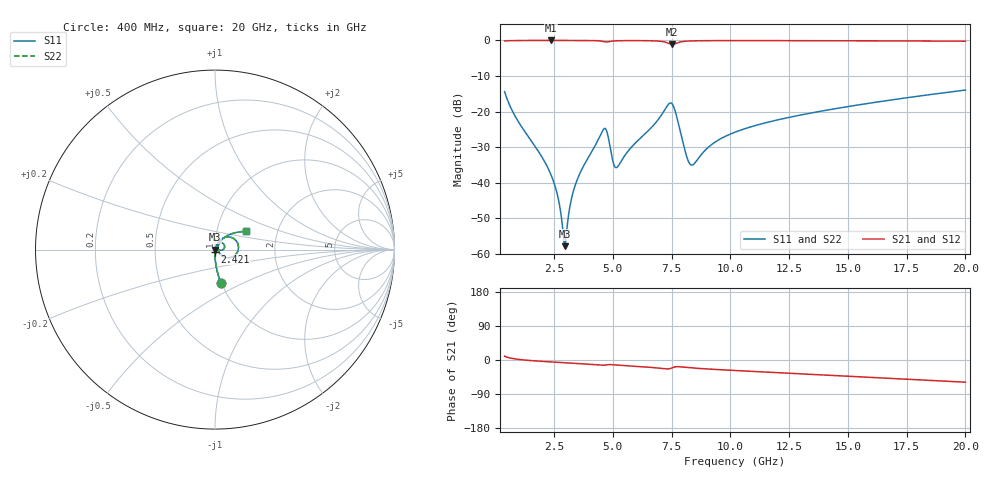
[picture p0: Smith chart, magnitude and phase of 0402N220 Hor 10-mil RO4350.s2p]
# GHz S MA R 50
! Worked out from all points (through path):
!   1960 points, 400 MHz to 20 GHz, reference 50 ohm
!   highest |S21| = -0.01 dB at 2.371 GHz (marker M1); lowest = -1.1 dB at 7.534 GHz (marker M2)
!   group delay of S21, straight-line fit = 8.43 ps
!   lowest |S11| = -57.9 dB at 2.961 GHz (marker M3), VSWR 1.00, Z = 50.1 - j0.0167 ohm
!   |S11| at or under -10 dB: start of sweep to end of sweep
!   |S22| runs from -57.9 to -14.0 dB; largest |S21 - S12| = 0
!   S11 on the Smith chart (normalised r, x): 400 MHz: 0.99, -0.39; 2.421 GHz: 1.00, -0.02; 20 GHz: 1.38, +0.29
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0.4  0.1906 -79.8  0.9811 10.0  0.9811 10.0  0.1906 -79.8
0.8702399  0.08333 -86.9  0.9958 2.6  0.9958 2.6  0.08333 -86.9
2.371006  0.0129 -90.3  0.9987 -5.1  0.9987 -5.1  0.0129 -90.3
2.421031  0.01173 -90.0  0.9987 -5.3  0.9987 -5.3  0.01173 -90.0
2.681164  0.005978 -85.0  0.9987 -6.3  0.9987 -6.3  0.005978 -85.0
2.901276  0.001758 -51.9  0.9986 -7.1  0.9986 -7.1  0.001758 -51.9
2.961307  0.001275 -7.5  0.9986 -7.3  0.9986 -7.3  0.001275 -7.5
3.28147  0.006687 68.8  0.9984 -8.4  0.9984 -8.4  0.006687 68.8
3.671669  0.01505 72.5  0.9977 -9.9  0.9977 -9.9  0.01505 72.5
4.622154  0.05698 35.3  0.9615 -13.8  0.9615 -13.8  0.05698 35.3
4.752221  0.05172 8.0  0.9512 -12.7  0.9512 -12.7  0.05172 8.0
5.022358  0.01909 3.9  0.9815 -12.6  0.9815 -12.6  0.01909 3.9
5.16243  0.01628 30.0  0.9879 -13.3  0.9879 -13.3  0.01628 30.0
6.943338  0.07774 55.2  0.9787 -21.3  0.9787 -21.3  0.07774 55.2
7.53364  0.127 -4.3  0.877 -20.4  0.877 -20.4  0.127 -4.3
8.143951  0.0233 -26.4  0.9765 -19.7  0.9765 -19.7  0.0233 -26.4
8.334048  0.01768 3.7  0.9835 -20.7  0.9835 -20.7  0.01768 3.7
9.244513  0.03505 54.6  0.9924 -24.5  0.9924 -24.5  0.03505 54.6
10.205  0.05124 57.1  0.9936 -27.7  0.9936 -27.7  0.05124 57.1
13.46667  0.0957 50.0  0.9913 -37.9  0.9913 -37.9  0.0957 50.0
16.73834  0.1436 40.5  0.9854 -48.1  0.9854 -48.1  0.1436 40.5
20  0.2003 30.4  0.9752 -58.6  0.9752 -58.6  0.2003 30.4
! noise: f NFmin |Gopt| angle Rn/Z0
0.4  0.001223  0.7799  1.331  0.001138
2.571  0.004473  0.6432  6.368  0.002365
4.752  0.03979  0.914  11.65  0.1009
6.933  0.02858  0.8337  16.88  0.03551
9.104  0.02091  0.7221  22.07  0.01438
11.29  0.0174  0.6159  26.87  0.007999
13.47  0.01805  0.5749  31.53  0.007173
15.64  0.01939  0.5533  36.04  0.00708
17.82  0.02096  0.5409  40.4  0.00722
20  0.02267  0.5342  44.6  0.007472
